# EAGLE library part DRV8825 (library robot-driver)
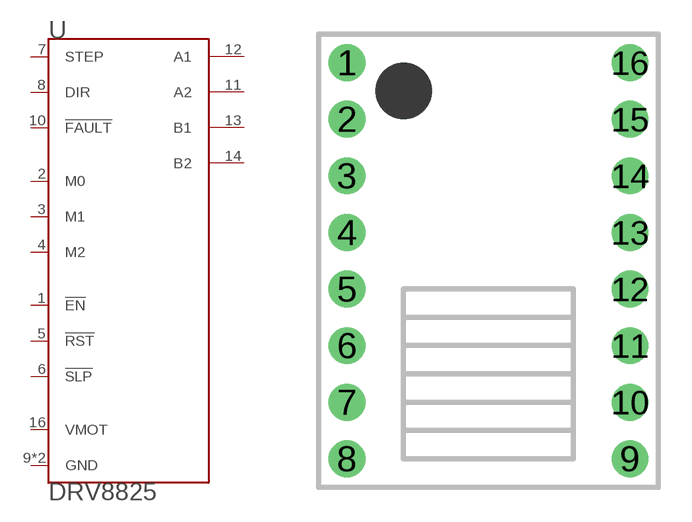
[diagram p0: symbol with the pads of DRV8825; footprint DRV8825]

Designator prefix -

## DRV8825  [DRV8825]
1  !EN
2  M0
3  M1
4  M2
5  !RST
6  !SLP
7  STEP
8  DIR
9  GND  pwr
10  !FAULT
11  A2
12  A1
13  B1
14  B2
15  GND  pwr
16  VMOT  pwr

## Footprint DRV8825 (pad centres in mm)
drill 0.762 pad 1.651: 1 -6.35,8.89; 2 -6.35,6.35; 3 -6.35,3.81; 4 -6.35,1.27; 5 -6.35,-1.27; 6 -6.35,-3.81; 7 -6.35,-6.35; 8 -6.35,-8.89; 9 6.35,-8.89; 10 6.35,-6.35; 11 6.35,-3.81; 12 6.35,-1.27; 13 6.35,1.27; 14 6.35,3.81; 15 6.35,6.35; 16 6.35,8.89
